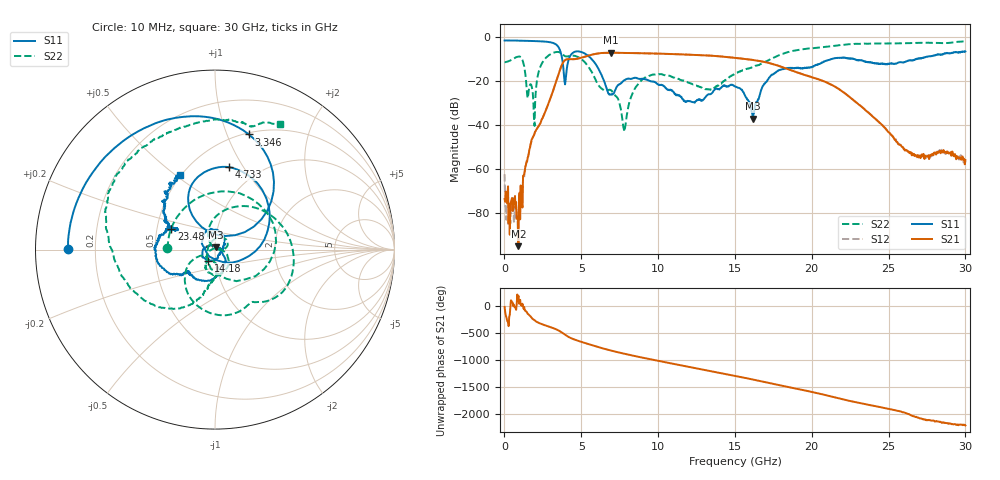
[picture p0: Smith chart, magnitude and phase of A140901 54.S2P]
!  2-Port S-parameters saved by WinCal
! VAR MeasName=S-Parameters (CALIBRATED_DATA) read from VNA (N5244A)
! VAR MeasDate=11/3/2014 9:36:08 AM
! VAR NAME=A140901 54
! VAR FILENAME=A140901 54.S2P
! VAR DATE=11/3/2014 9:36:08 AM
! VAR PHYS_PORTS=1,2
# Hz S RI R 50
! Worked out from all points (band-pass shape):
!   801 points, 10 MHz to 30 GHz, reference 50 ohm
!   highest |S21| = -7.24 dB at 6.908 GHz (marker M1); lowest = -94.9 dB at 909.7 MHz (marker M2)
!   |S21| within 3 dB of the highest: 4.071 GHz to 15.82 GHz (11.75 GHz wide, 118 % of centre)
!   lowest |S11| = -37.2 dB at 16.17 GHz (marker M3), VSWR 1.03, Z = 50.4 + j1.32 ohm
!   |S11| at or under -10 dB: 3.753 GHz to 4.197 GHz (444.7 MHz wide, 11.2 % of centre); 5.653 GHz to 21.36 GHz (15.7 GHz wide, 116 % of centre); 22.7 GHz to 26.84 GHz (4.137 GHz wide, 16.7 % of centre)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
!   |S22| runs from -43.0 to -2.1 dB; largest |S21 - S12| = 0.0023
!   S11 on the Smith chart (normalised r, x): 10 MHz: 0.10, +0.00; 3.346 GHz: 0.52, +1.20; 4.733 GHz: 0.74, +0.87; 14.18 GHz: 0.92, -0.12; 23.48 GHz: 0.59, +0.15; 30 GHz: 0.49, +0.52
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1e7  -0.8193 0.00459  0.000199 -6.75e-05  -0.000584 -0.000496  -0.2647 0.00619
2.34925e8  -0.8161 0.0763  9.34e-05 0.000397  -4.89e-05 3.04e-05  -0.2263 0.1563
9.097e8  -0.7592 0.2908  -1.79e-05 -2.54e-06  -0.000114 1.55e-05  0.2729 0.225
1.921862e9  -0.5493 0.5746  -0.00134 0.00571  -0.00122 0.00566  0.0142 0.000286
2.4092e9  -0.3786 0.6836  0.0116 0.00556  0.0115 0.00571  0.0705 0.2271
3.346388e9  0.1885 0.6418  0.0295 -0.0877  0.0294 -0.0878  0.4359 -0.0997
3.946188e9  0.00981 0.0825  -0.2939 -0.0204  -0.2932 -0.0204  0.2133 -0.2914
4.733425e9  0.0801 0.4587  0.0592 0.3099  0.0591 0.3096  -0.0314 -0.3518
5.033325e9  0.2173 0.3883  0.211 0.2603  0.2103 0.2603  -0.1325 -0.2762
6.9077e9  -0.0334 -0.0361  -0.1179 -0.418  -0.1172 -0.418  -0.0478 -0.0387
7.8074e9  -0.0645 0.0804  -0.4163 -0.0973  -0.4153 -0.0977  -0.000778 0.00701
8.594638e9  -0.02 0.1146  -0.3437 0.2482  -0.3442 0.2478  0.0681 -0.032
1.001916e10  0.0469 0.0672  0.201 0.3626  0.2 0.3613  0.00241 -0.1401
1.241836e10  0.0259 -0.0218  0.1192 -0.367  0.1188 -0.3671  -0.0449 -0.0665
1.418028e10  -0.0368 -0.0638  -0.3487 -0.0592  -0.3492 -0.0592  0.0131 -0.0918
1.5005e10  -0.0704 -0.0252  -0.2652 0.1982  -0.2639 0.1987  0.00766 -0.1448
1.616711e10  0.00439 0.0131  0.0717 0.2885  0.0713 0.287  -0.0376 -0.2008
1.747918e10  0.0245 -0.1372  0.2383 -0.016  0.2382 -0.0152  -0.1269 -0.3031
2.002832e10  -0.1637 -0.1263  -0.1095 -0.0491  -0.1092 -0.0504  -0.5336 -0.1143
2.347718e10  -0.2438 0.1148  0.0204 -0.00792  0.0206 -0.00786  -0.4835 0.502
2.501416e10  -0.2099 0.1144  -0.00211 -0.00651  -0.00206 -0.00642  -0.2662 0.6511
3e10  -0.1976 0.4167  0.000898 -0.00131  0.000802 -0.00118  0.3616 0.7
